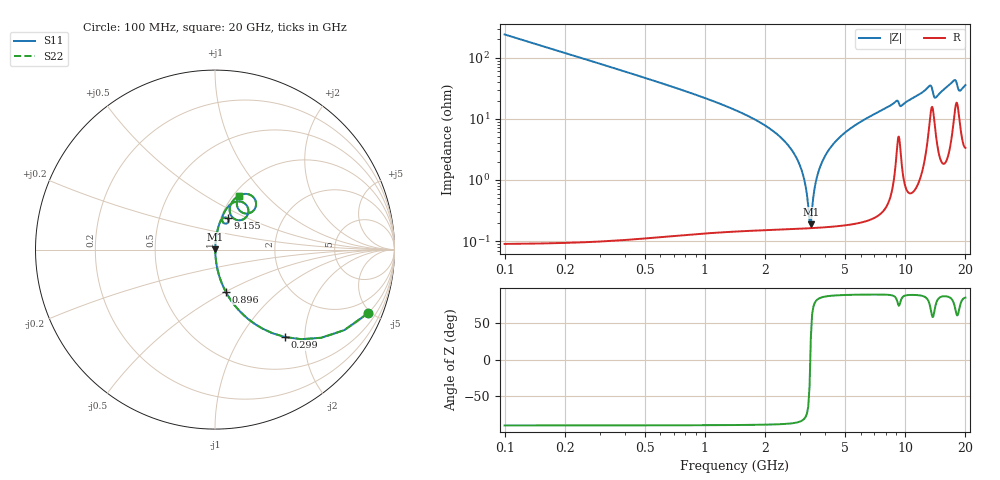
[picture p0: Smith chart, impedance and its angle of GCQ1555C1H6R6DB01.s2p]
!Murata Part Number: GCQ1555C1H6R6DB01
!These Parameters are Measured in Series Mode Connection
!Data Generated on Mar 13, 2026
!  o--ll--o
!Port1  Port2
!  o------o
!Operation Temp=25[degC], DC Bias Voltage=0[V]
!Freq. Start=100[MHz] Stop=20[GHz] 401[Steps]
# Hz S RI R 50
!Freq.(Hz) S11(Real) S11(Imag) S21(Real) S21(Imag) S12(Real) S12(Imag) S22(Real) S22(Imag)
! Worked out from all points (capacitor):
!   401 points, 100 MHz to 20 GHz, reference 50 ohm
!   read as one part in series: C = 6.6 pF near 199.5 MHz
!   lowest |Z| = 189 mohm at 3.384 GHz (marker M1)
!   series resonance near 3.361 GHz, so ESL is about 340 pH
!   S11 on the Smith chart (normalised r, x): 100 MHz: 1.00, -4.82; 299 MHz: 1.00, -1.60; 896 MHz: 1.00, -0.50; 9.155 GHz: 1.08, +0.39; 20 GHz: 1.07, +0.71
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1e8  0.8529 -0.354  0.1471 0.354  0.1471 0.354  0.8529 -0.354
2.99e8  0.3903 -0.4872  0.6097 0.4872  0.6097 0.4872  0.3903 -0.4872
5.4775e8  0.1557 -0.3612  0.8443 0.3612  0.8443 0.3612  0.1557 -0.3612
8.96e8  0.0598 -0.2346  0.9402 0.2346  0.9402 0.2346  0.0598 -0.2346
2.73675e9  0.00245 -0.0296  0.9975 0.0296  0.9975 0.0296  0.00245 -0.0296
3.03525e9  0.00181 -0.0147  0.9982 0.0147  0.9982 0.0147  0.00181 -0.0147
3.284e9  0.00163 -0.00333  0.9984 0.00333  0.9984 0.00333  0.00163 -0.00333
3.3835e9  0.00162 0.000956  0.9984 -0.000956  0.9984 -0.000956  0.00162 0.000956
3.43325e9  0.00164 0.00305  0.9984 -0.00305  0.9984 -0.00305  0.00164 0.00305
3.5825e9  0.00173 0.00918  0.9983 -0.00918  0.9983 -0.00918  0.00173 0.00918
3.73175e9  0.00188 0.0151  0.9981 -0.0151  0.9981 -0.0151  0.00188 0.0151
4.22925e9  0.00282 0.0334  0.9972 -0.0334  0.9972 -0.0334  0.00282 0.0334
5.1745e9  0.00598 0.0643  0.994 -0.0643  0.994 -0.0643  0.00598 0.0643
6.7665e9  0.0146 0.1104  0.9854 -0.1104  0.9854 -0.1104  0.0146 0.1104
9.1545e9  0.0699 0.1749  0.9301 -0.1749  0.9301 -0.1749  0.0699 0.1749
1.005e10  0.0402 0.177  0.9598 -0.177  0.9598 -0.177  0.0402 0.177
1.338325e10  0.1775 0.2443  0.8225 -0.2443  0.8225 -0.2443  0.1775 0.2443
1.407975e10  0.1049 0.173  0.8951 -0.173  0.8951 -0.173  0.1049 0.173
1.67165e10  0.1388 0.3038  0.8612 -0.3038  0.8612 -0.3038  0.1388 0.3038
1.77115e10  0.2202 0.2836  0.7798 -0.2836  0.7798 -0.2836  0.2202 0.2836
1.865675e10  0.1431 0.2119  0.8569 -0.2119  0.8569 -0.2119  0.1431 0.2119
2e10  0.135 0.2978  0.865 -0.2978  0.865 -0.2978  0.135 0.2978
